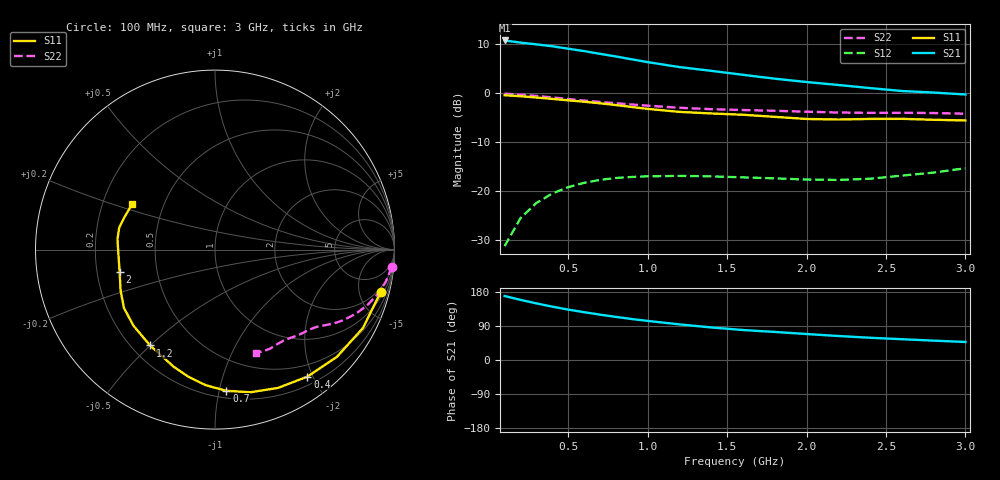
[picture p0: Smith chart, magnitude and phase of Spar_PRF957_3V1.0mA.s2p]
! Filename:  PRF957B.S2P  Version:  3.0
! NXP part #:  PRF957  Date:  Nov 1998
! Bias condition:  Vce=3V, Ic=1.0mA
#  MHz  S  MA  R 50
! Freq  S11  S21  S12  S22
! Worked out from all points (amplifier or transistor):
!   20 points, 100 MHz to 3 GHz, reference 50 ohm
!   highest |S21| = 10.8 dB at 100 MHz (marker M1)
!   |S21| within 3 dB of that: start of sweep to 749.9 MHz
!   unconditionally stable (mu >= 1): 2.034 GHz to end of sweep
!   at 400 MHz: K = 0.15, MSG = 15.1 dB, |S12| = -20.5 dB
!   at 1.2 GHz: K = 0.51, MSG = 11.1 dB, |S12| = -16.9 dB
!   at 3 GHz: K = 1.17, MAG = 5.0 dB, |S12| = -15.3 dB
!   S11 on the Smith chart (normalised r, x): 100 MHz: 1.47, -7.71; 400 MHz: 0.32, -1.92; 700 MHz: 0.25, -1.05; 1.2 GHz: 0.27, -0.50; 2 GHz: 0.30, -0.11; 3 GHz: 0.33, +0.23
100  0.954 -14.3  3.468 168.9  0.02727 81.3  0.9907 -5.5
200  0.9325 -28.0  3.297 158.7  0.05275 73.6  0.9681 -10.7
300  0.9048 -41.3  3.164 149.4  0.07541 66.5  0.9387 -15.4
400  0.8752 -54.0  3.025 140.7  0.09423 60.2  0.9064 -19.6
500  0.8468 -65.5  2.857 133.1  0.1094 55.0  0.8725 -23.3
600  0.8189 -76.0  2.7 126.1  0.1212 50.5  0.8418 -26.3
700  0.7894 -85.4  2.532 119.8  0.1299 46.7  0.815 -28.9
800  0.7572 -93.9  2.381 113.8  0.1359 43.5  0.7905 -30.9
900  0.7236 -101.8  2.224 108.2  0.1392 41.0  0.7676 -32.7
1000  0.6922 -109.4  2.082 103.2  0.1414 39.0  0.7464 -34.3
1200  0.645 -124.1  1.853 94.0  0.1428 36.1  0.7104 -37.4
1400  0.6213 -137.0  1.696 85.9  0.1412 34.7  0.6871 -40.6
1600  0.6026 -147.3  1.544 79.1  0.1379 35.7  0.6738 -43.7
1800  0.5736 -156.5  1.41 74.1  0.1348 38.5  0.6619 -46.4
2000  0.5457 -166.8  1.303 68.6  0.131 42.6  0.6477 -49.3
2200  0.5389 -177.5  1.215 63.3  0.1298 48.1  0.6351 -53.0
2400  0.5465 173.8  1.13 58.7  0.1336 54.5  0.6303 -57.2
2600  0.5475 167.0  1.054 54.9  0.1437 61.2  0.6313 -61.0
2800  0.5353 160.0  1.017 51.1  0.1544 67.6  0.6274 -64.5
3000  0.5267 151.4  0.9715 47.6  0.1711 73.0  0.6173 -68.5
